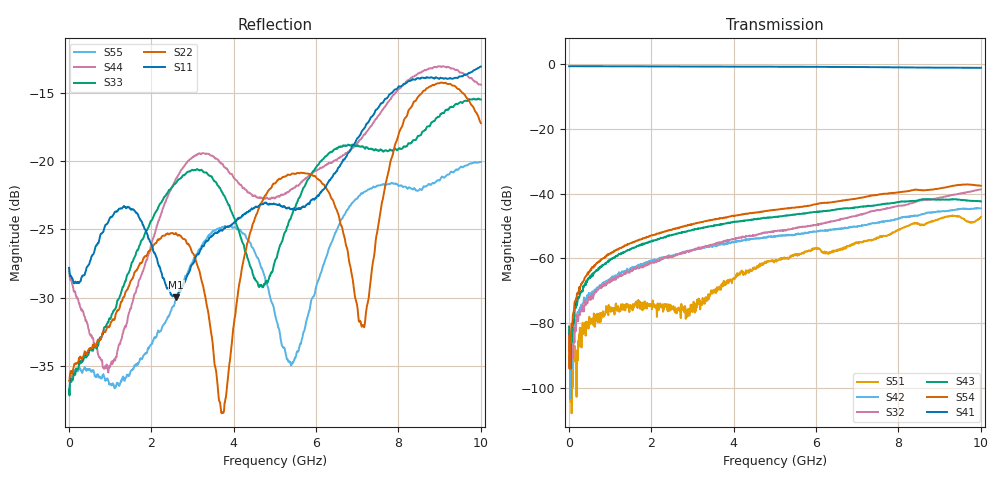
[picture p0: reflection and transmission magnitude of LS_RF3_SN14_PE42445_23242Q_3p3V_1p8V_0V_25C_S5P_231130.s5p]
!Keysight Technologies,M9804A,MY58100185,A.15.10.06
!Date: Thursday, November 30, 2023 12:04:58
!Correction: S11(Cdelta 6-Port  )
!S12(Cdelta 6-Port  )
!S13(Cdelta 6-Port  )
!S15(Cdelta 6-Port  )
!S16(Cdelta 6-Port  )
!S21(Cdelta 6-Port  )
!S22(Cdelta 6-Port  )
!S23(Cdelta 6-Port  )
!S25(Cdelta 6-Port  )
!S26(Cdelta 6-Port  )
!S31(Cdelta 6-Port  )
!S32(Cdelta 6-Port  )
!S33(Cdelta 6-Port  )
!S35(Cdelta 6-Port  )
!S36(Cdelta 6-Port  )
!S51(Cdelta 6-Port  )
!S52(Cdelta 6-Port  )
!S53(Cdelta 6-Port  )
!S55(Cdelta 6-Port  )
!S56(Cdelta 6-Port  )
!S61(Cdelta 6-Port  )
!S62(Cdelta 6-Port  )
!S63(Cdelta 6-Port  )
!S65(Cdelta 6-Port  )
!S66(Cdelta 6-Port  )
!S5P File: Measurements: <S11,S12,S13,S15,S16>,
!<S21,S22,S23,S25,S26>,
!<S31,S32,S33,S35,S36>,
!<S51,S52,S53,S55,S56>,
!<S61,S62,S63,S65,S66>:
# Hz S  dB  R 50
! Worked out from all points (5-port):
!   1000 points, 10 MHz to 10 GHz, reference 50 ohm
!   strongest paths, dB at 10 MHz, 2.51 GHz, 5.01 GHz, 7.51 GHz, 10 GHz:
!     S41: -0.6, -0.7, -0.7, -0.9, -1.1
!     S54: -83.8, -51.2, -45.0, -40.3, -37.5
!     S43: -81.1, -52.7, -47.1, -43.5, -42.4
!     S32: -91.6, -59.5, -51.5, -45.0, -38.7
!     S42: -82.5, -59.3, -53.4, -48.9, -44.5
!     S51: -82.3, -75.5, -60.7, -53.6, -47.2
!   lowest |S11| = -30.0 dB at 2.61 GHz (marker M1), VSWR 1.07, Z = 48 - j2.34 ohm
!   |S11| at or under -10 dB: start of sweep to end of sweep
